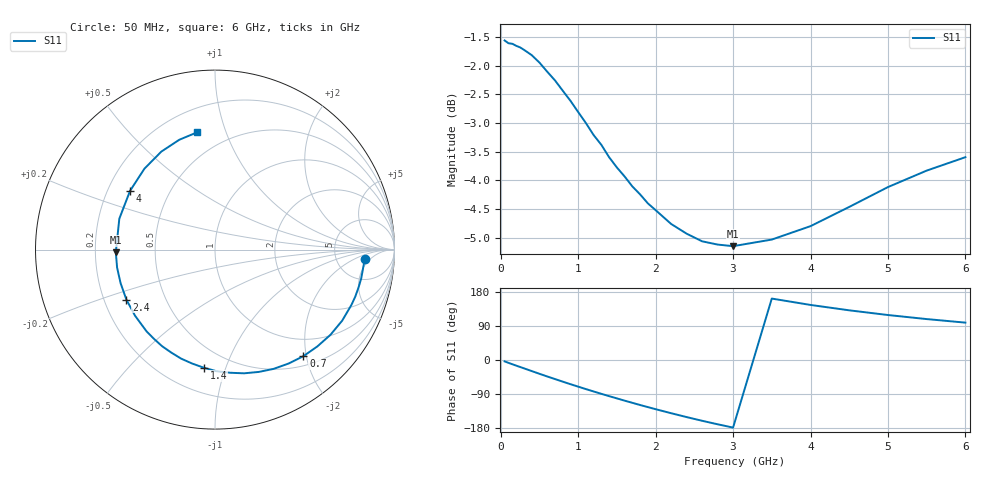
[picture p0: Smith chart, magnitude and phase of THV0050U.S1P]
! SIEMENS Discrete & RF Semiconductors
! BAS70
! Si Schottky Diode in SOT23
! IF = 0.05 mA
! S-Parameters:  February  1997
# GHz  S  MA  R  50
!  f  S11
! GHz  MAG  ANG
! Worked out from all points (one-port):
!   34 points, 50 MHz to 6 GHz, reference 50 ohm
!   lowest |S11| = -5.1 dB at 3 GHz (marker M1), VSWR 3.47, Z = 14.4 - j0.64 ohm
!   |S11| at or under -10 dB: nowhere
!   S11 on the Smith chart (normalised r, x): 50 MHz: 10, -4; 700 MHz: 0.66, -1.95; 1.4 GHz: 0.36, -0.84; 2.4 GHz: 0.29, -0.24; 4 GHz: 0.29, +0.29; 6 GHz: 0.34, +0.80
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0.05  0.8359 -3.7
0.15  0.8304 -11.2
0.25  0.8243 -18.4
0.3  0.8204 -22.0
0.4  0.8116 -29.2
0.5  0.7995 -36.4
0.6  0.7851 -43.4
0.7  0.7715 -50.3
0.8  0.7557 -57.1
0.9  0.7405 -63.8
1  0.7239 -70.3
1.1  0.708 -76.8
1.3  0.6776 -89.3
1.4  0.661 -95.4
1.6  0.6359 -107.3
1.8  0.6135 -118.8
2  0.5944 -129.8
2.2  0.5781 -140.4
2.4  0.5669 -150.6
2.6  0.5583 -160.4
2.8  0.5546 -169.6
3  0.5528 -178.4
3.5  0.5602 162.1
4  0.5755 145.3
4.5  0.5982 131.1
5  0.6226 118.7
5.5  0.6435 108.0
6  0.6611 98.6
